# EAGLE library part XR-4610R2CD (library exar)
R/W PREAMPLIFIER
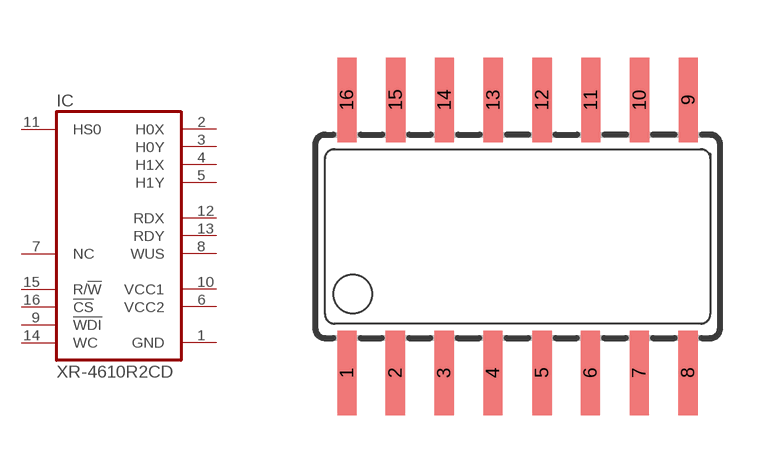
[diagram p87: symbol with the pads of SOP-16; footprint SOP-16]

Designator prefix IC

## XR-4610R2CD (OC_FARNELL: unknown; OC_NEWARK: unknown)  [SOP-16]
1  GND  pwr
2  H0X
3  H0Y
4  H1X
5  H1Y
6  VCC2  pwr
7  NC  nc
8  WUS  out
9  !WDI  in
10  VCC1  pwr
11  HS0  in
12  RDX  out
13  RDY  out
14  WC  in
15  R/!W  in
16  !CS  in

## Footprint SOP-16 (pad centres in mm)
Small Outline Package
smd 0.5 x 2.2: 1 -4.445,-3.55; 2 -3.185,-3.55; 3 -1.915,-3.55; 4 -0.645,-3.55; 5 0.635,-3.55; 6 1.895,-3.55; 7 3.165,-3.55; 8 4.435,-3.55; 9 4.445,3.55; 10 3.175,3.55; 11 1.905,3.55; 12 0.635,3.55; 13 -0.635,3.55; 14 -1.905,3.55; 15 -3.175,3.55; 16 -4.445,3.55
